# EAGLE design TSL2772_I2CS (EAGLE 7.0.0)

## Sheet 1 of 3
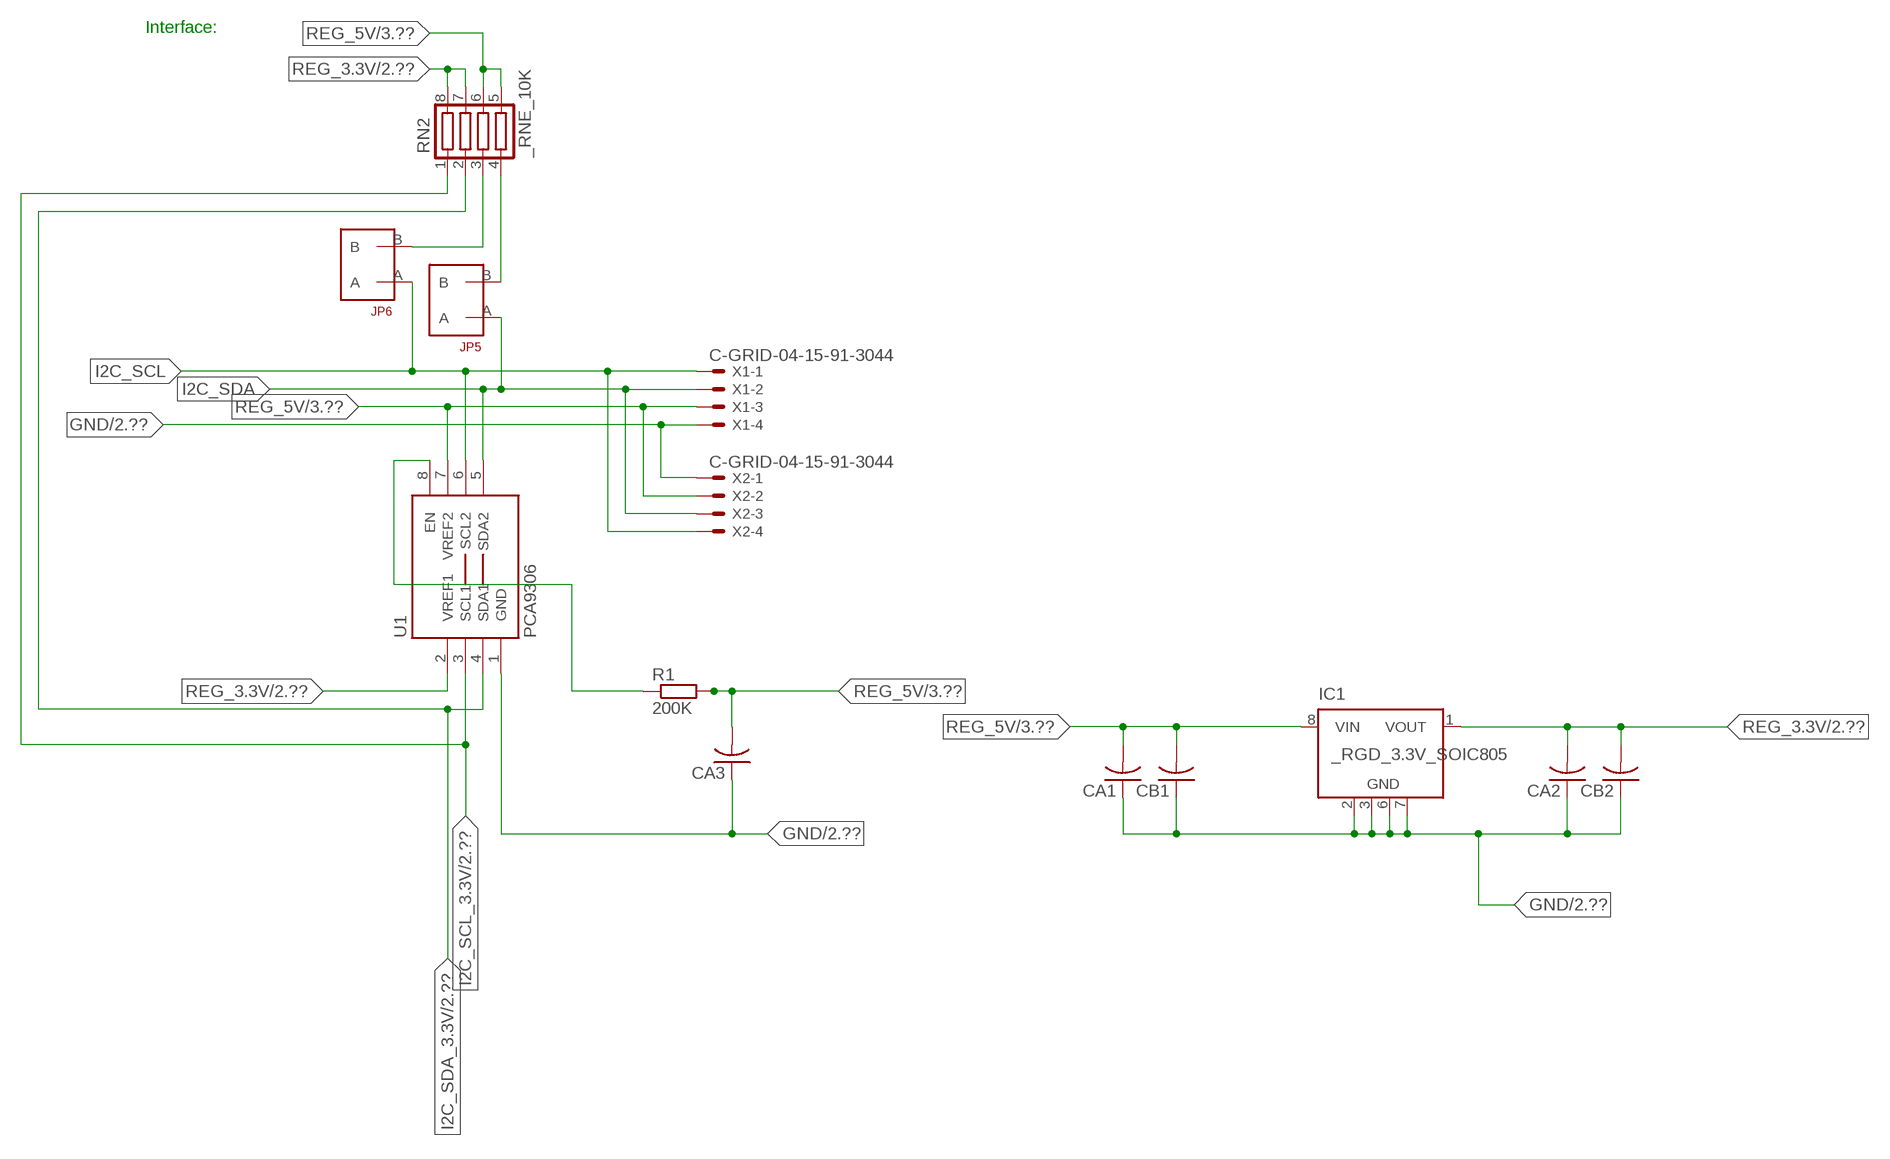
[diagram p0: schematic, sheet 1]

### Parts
CA1  CC1206KRX7R9BB104  [.1UF]
CA2  CC1206KRX7R9BB104  [.1UF]
CA3  CC1206KRX7R9BB104  [.1UF]
CB1  TMK316F106ZL-TC1206K  [TMK316F106ZL-T]
CB2  TMK316F106ZL-TC1206K  [TMK316F106ZL-T]
IC1  _RGD_3.3V_SOIC805  [_RGC_3.3V_SOIC8]
JP5  JUMPER_1X2_2MM  [JUMPER_1X2_2MM]
JP6  JUMPER_1X2_2MM  [JUMPER_1X2_2MM]
R1  200K  RESISTOR_SMT-0603  [R603]
RN2  _RNE_10K  [RNE]
U1  PCA9306  PCA9306_NCD  [PSOP-8]
X1  C-GRID-04-15-91-3044  [15-91-04]
X2  C-GRID-04-15-91-3044  [15-91-04]

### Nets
GND: CA1.1 CA2.1 CA3.1 CB1.1 CB2.1 IC1.2(GND) IC1.3(GND) IC1.6(GND) IC1.7(GND) U1.1(GND) X1.4 X2.1 ; also sheet 2,3
I2C_SCL: JP6.A U1.6(SCL2) X1.1 X2.4
I2C_SCL_3.3V: RN2.1 U1.3(SCL1) ; also sheet 2
I2C_SDA: JP5.A U1.5(SDA2) X1.2 X2.3
I2C_SDA_3.3V: RN2.2 U1.4(SDA1) ; also sheet 2
N$1: JP6.B RN2.3
N$2: JP5.B RN2.4
N$24: R1.1 U1.8(EN)
REG_3.3V: CA2.2 CB2.2 IC1.1(VOUT) RN2.7 RN2.8 U1.2(VREF1) ; also sheet 2
REG_5V: CA1.2 CA3.2 CB1.2 IC1.8(VIN) R1.2 RN2.5 RN2.6 U1.7(VREF2) X1.3 X2.2 ; also sheet 3
Unconnected: IC1.4(NC) IC1.5(NC)

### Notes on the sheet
- Interface:

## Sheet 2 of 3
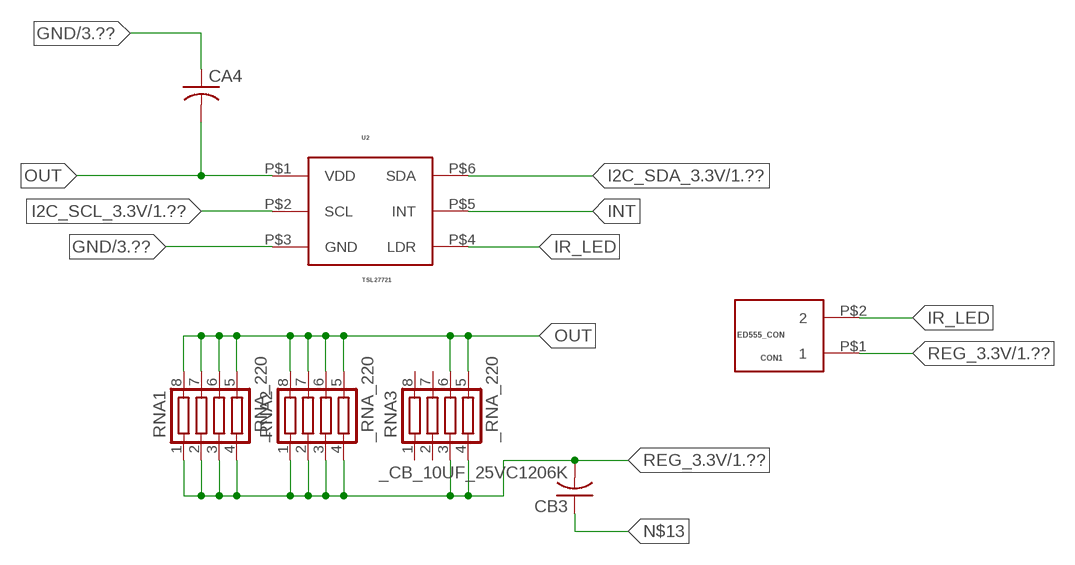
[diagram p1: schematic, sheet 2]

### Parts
CA4  _CA_.10UF_50VC1206K  [_CA_.1UF_50V]
CB3  _CB_10UF_25VC1206K  [_CB_10UF_25V]
CON1  ED555_CON  [ED555_CON]
RNA1  _RNA_220  [RNA]
RNA2  _RNA_220  [RNA]
RNA3  _RNA_220  [RNA]
U2  TSL27721  TSL2771  [TSL2771]

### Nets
GND: CA4.1 U2.P$3(GND) ; also sheet 1,3
I2C_SCL_3.3V: U2.P$2(SCL) ; also sheet 1
I2C_SDA_3.3V: U2.P$6(SDA) ; also sheet 1
INT: U2.P$5(INT)
IR_LED: CON1.P$2 U2.P$4(LDR)
N$13: CB3.1
OUT: CA4.2 RNA1.5 RNA1.6 RNA1.7 RNA1.8 RNA2.5 RNA2.6 RNA2.7 RNA2.8 RNA3.5 RNA3.6 U2.P$1(VDD)
REG_3.3V: CB3.2 CON1.P$1 RNA1.1 RNA1.2 RNA1.3 RNA1.4 RNA2.1 RNA2.2 RNA2.3 RNA2.4 RNA3.3 RNA3.4 ; also sheet 1
Unconnected: RNA3.1 RNA3.2 RNA3.7 RNA3.8

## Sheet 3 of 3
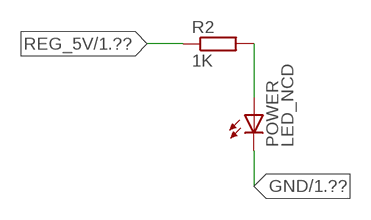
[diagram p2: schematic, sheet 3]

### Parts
POWER  LED_NCD  [CHIPLED_0603]
R2  1K  RESISTOR_SMT-0402  [R402]

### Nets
GND: POWER.C ; also sheet 1,2
N$4: POWER.A R2.2
REG_5V: R2.1 ; also sheet 1

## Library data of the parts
CA1-CA3 = NCD_ULTIMATE_LIBRARY:CC1206KRX7R9BB104: Capacitor CA .1uF 50V SMT C1206K CC1206KRX7R9BB104
CA4 = NCD_ULTIMATE_LIBRARY:_CA_.10UF_50V: Capacitor .1uF SMT
CB1 CB2 = NCD_ULTIMATE_LIBRARY:TMK316F106ZL-T: Capacitor CB 10uF SMT 1206 TMK316F106ZL-T
CB3 = NCD_ULTIMATE_LIBRARY:_CB_10UF_25V: Capacitor 10uF SMT
CON1 = NCD_ULTIMATE_bhaskar:ED555_CON: Digikey ED1514-ND/ ED555/2DS NCD CON
IC1 = NCD_ULTIMATE_LIBRARY:_RGD_3.3V_SOIC8: Regulator Linear 3.3V Chip Positive VOLTAGE REGULATOR Digikey 497-1199-2-ND/L78L33ACD13TR
JP5 JP6 = NCD_ULTIMATE_CONNECTORS:JUMPER_1X2_2MM
POWER = NCD_ULTIMATE_LIBRARY:LED_NCD: LED Digikey 754-1132-2-ND/APT2012SRCPRV
R1 R2 = NCD_ULTIMATE_LIBRARY:RESISTOR_SMT: NCD Resistor
RN2 = NCD_ULTIMATE_LIBRARY:_RNE_10K: Resistor Array RNE SMT 10K x 4 Single Resistor Source: http://www.ctscorp.com/components/Datasheets/CTSChipArrayDs.pdf Digikey 742C083103JPTR-ND/742C083103JP; OC_FARNELL: unknown; OC_NEWARK: unknown
RNA1-RNA3 = NCD_ULTIMATE_LIBRARY:_RNA_220: Resistor Array RNA SMT 220 x 4 Single Resistor Source: http://www.ctscorp.com/components/Datasheets/CTSChipArrayDs.pdf Digikey 742C083221JPTR-ND/742C083221JP; OC_FARNELL: unknown; OC_NEWARK: unknown
U1 = NCD_ULTIMATE_LIBRARY:PCA9306_NCD: NCD Bidirectional I2C level shifter. NOT compatible with all available part number pinout schemes- DOUBLE CHECK!!!; PROD_ID: IC-10023
U2 = NCD_ULTIMATE_bhaskar:TSL2771
X1 X2 = NCD_ULTIMATE_CONNECTORS:C-GRID-04: CONNECTOR 4-Pos I2C wire to board 2.54 mm (0.100") pitch header Digikey WM1342-ND/0015912045; OC_FARNELL: unknown; OC_NEWARK: unknown

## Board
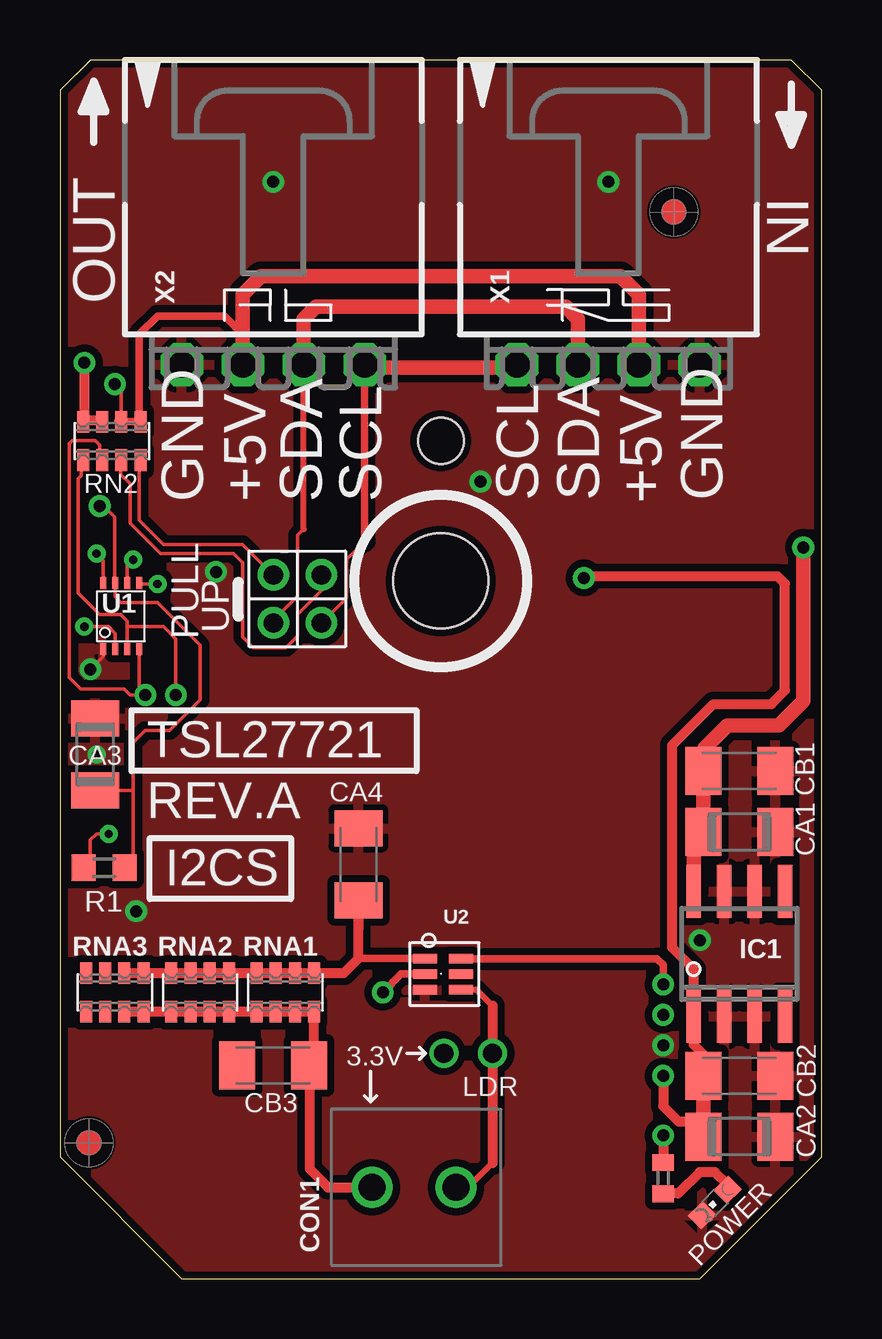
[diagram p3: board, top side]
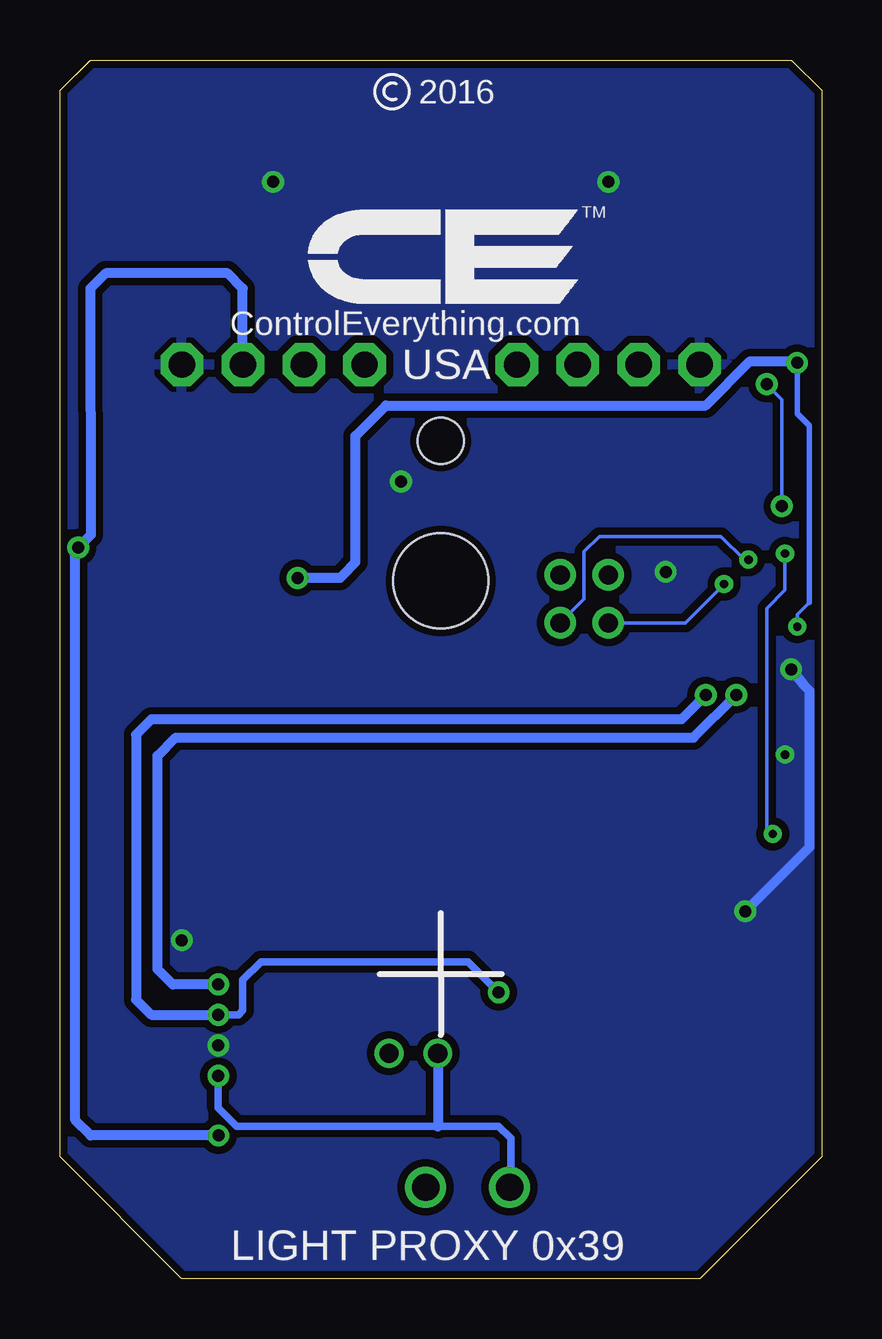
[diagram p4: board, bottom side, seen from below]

Size 31.75 x 50.8 mm. Coordinates in mm from the lower left corner, seen from the top.
Outline: 48 segments
Copper layers (1*16): Top 0.035mm / dielectric 1.5mm / Bottom 0.035mm
Design rules "default": minimum track width 5mil, minimum drill 24mil, track to track 5mil, track to pad 5mil, pad to pad 5mil, via to via 5mil, smd to smd 5mil, copper to edge 10mil, drill to drill 8mil, minimum pad ring 10mil, minimum via ring 8mil, stop-mask expansion 2mil, vias tented up to drill 0mil, thermal gap 10mil
Holes 3.96 mm at 15.88,29.08
Holes 1.91 mm at 15.88,34.93

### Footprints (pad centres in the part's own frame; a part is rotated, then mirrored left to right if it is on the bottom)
.1UF = smd 1.5 x 2: 1 -1.5,0; 2 1.5,0
_CA_.1UF_50V = smd 1.5 x 2: 1 -1.5,0; 2 1.5,0
TMK316F106ZL-T = smd 1.5 x 2: 1 -1.5,0; 2 1.5,0
_CB_10UF_25V = smd 1.5 x 2: 1 -1.5,0; 2 1.5,0
ED555_CON = drill 1.143: P$1 0,3.5; P$2 0,0
_RGC_3.3V_SOIC8 = smd 0.6 x 2.2: 1 -1.905,-2.6; 2 -0.635,-2.6; 3 0.635,-2.6; 4 1.905,-2.6; 5 1.905,2.6; 6 0.635,2.6; 7 -0.635,2.6; 8 -1.905,2.6
JUMPER_1X2_2MM = drill 0.8: A 0,2; B 0,0
CHIPLED_0603 = smd 0.8 x 0.876: A 0,-0.75; C 0,0.75
R603 = smd 1 x 1.1: 1 -0.85,0; 2 0.85,0
R402 = smd 0.7 x 0.9: 1 -0.65,0; 2 0.65,0
RNE = smd 0.5 x 0.9: 1 -1.2,-0.8; 2 -0.4,-0.8; 3 0.4,-0.8; 4 1.2,-0.8; 5 1.2,0.8; 6 0.4,0.8; 7 -0.4,0.8; 8 -1.2,0.8
RNA = smd 0.5 x 0.9: 1 -1.2,-0.8; 2 -0.4,-0.8; 3 0.4,-0.8; 4 1.2,-0.8; 5 1.2,0.8; 6 0.4,0.8; 7 -0.4,0.8; 8 -1.2,0.8
PSOP-8 = smd 0.25 x 0.5: 1 -0.73,-1.37; 2 -0.23,-1.37; 3 0.27,-1.37; 4 0.77,-1.37; 5 0.77,1.38; 6 0.27,1.38; 7 -0.23,1.38; 8 -0.73,1.38
TSL2771 = smd 1 x 0.4: P$1 -0.65,0.65; P$2 -0.65,0; P$3 -0.65,-0.65; P$4 0.85,-0.65; P$5 0.85,0; P$6 0.85,0.65
15-91-04 = drill 1.1 pad 1.778 octagon: 1 -3.81,-7.62; 2 -1.27,-7.62; 3 1.27,-7.62; 4 3.81,-7.62

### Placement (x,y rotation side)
CA1  28.32,18.62 180 top
CA2  28.32,5.92 180 top
CA3  1.46,21.86 270 top
CA4  12.45,17.27 270 top
CB1  28.32,21.16 180 top
CB2  28.32,8.46 180 top
CB3  8.89,8.89 0 top
CON1  16.51,3.81 90 top
IC1  28.32,13.54 0 top
JP5  8.89,29.34 180 top
JP6  10.9,29.34 180 top
POWER  27.3,3.18 135 top
R1  1.84,17.13 0 top
R2  25.15,4.19 270 top
RN2  2.16,34.93 0 top
RNA1  9.4,11.94 0 top
RNA2  5.84,11.94 0 top
RNA3  2.29,11.94 0 top
U1  2.54,27.61 0 top
U2  15.88,12.7 0 top
U$5  [VISION_REF10]  1.21,5.66 90 top
U$28  [VISION_REF10]  25.59,44.46 90 top
X1  22.86,45.72 0 top
X2  8.89,45.72 0 top

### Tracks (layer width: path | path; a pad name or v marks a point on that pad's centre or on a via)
GND  (via drill 0.35, 0.5)
  Top 0.152: CA3.1 1.52,23.42 1.52,23.62 | v1.27,25.4 1.81,25.94 U1.1
  Bottom 0.406: v1.27,25.4 0.76,24.77 0.51,24.51 0.51,17.99 v3.18,15.32
  other vias: 8.89,45.72 22.86,45.72 25.15,9.73 17.53,33.22 26.67,14.11 6.5,29.46 1.52,21.84
  pour Bottom (isolate 0.305): -0.64,5.08 -0.64,49.53 1.27,51.44 30.48,51.44 32.38,49.53 32.38,5.08 26.67,-0.63 5.08,-0.63
  pour Top (isolate 0.305): 4.45,-1.27 -1.27,4.45 -1.27,50.17 0.64,52.07 31.11,52.07 33.02,50.17 33.02,4.45 27.3,-1.27
I2C_SCL  (via drill 0.35)
  Top 0.152: 12.7,30.73 11.94,29.97 11.94,28.38 JP6.A | v3.05,29.97 2.81,29.73 U1.6
  Top 0.305: 12.7,30.73 X2.4
  Top 0.406: X2.4 12.7,37.97 | 19.05,37.97 X1.1
  Top 0.61: 12.7,37.97 19.05,37.97
  Bottom 0.152: JP6.A 9.91,28.33 9.91,30.3 9.27,30.94 4.19,30.94 3.23,29.97 v3.05,29.97
I2C_SCL_3.3V  (via drill 0.5)
  Top 0.152: RN2.1 0.89,34.07 0.89,33.48 0.77,33.35 0.77,28.59 1.67,27.69 2.54,27.69 2.81,27.42 2.81,27.18 | 2.81,27.18 U1.3 | v4.83,24.33 v4.83,24.34 4.83,26.67 4.32,27.18 2.81,27.18
  Top 0.305: U2.P$2 14.22,12.7 v13.46,11.94
  Bottom 0.305: v13.46,11.94 14.73,13.21 23.37,13.21 24.13,12.45 24.13,11.18 24.31,11 v25.15,11
  Bottom 0.406: v4.83,24.33 5.84,23.32 27.94,23.32 28.58,22.68 28.58,11.63 27.94,11 v25.15,11
I2C_SDA  (via drill 0.35)
  Top 0.152: JP5.A 8.89,27.44 9.91,28.45 9.91,30.99 10.16,31.24 | U1.5 3.34,28.96 v4.06,28.96
  Top 0.254: 10.16,31.24 10.16,31.25 X2.3
  Top 0.61: X2.3 10.16,40.01 10.67,40.51 21.09,40.51 21.59,40.01 X1.2
  Bottom 0.152: v4.06,28.96 5.68,27.34 JP5.A
I2C_SDA_3.3V  (via drill 0.5)
  Top 0.152: RN2.2 1.65,34.14 1.65,34.75 1.46,34.94 0.51,34.94 0.38,34.81 0.38,26.37 0.38,26.36 0.38,25.07 0.86,24.59 2.67,24.59 2.92,24.33 v3.56,24.33 3.31,24.58 U1.4
  Top 0.305: U2.P$6 17.12,13.34 24.89,13.34 25.15,13.08 v25.15,12.27
  Bottom 0.406: v25.15,12.27 27.05,12.27 27.69,12.9 27.69,21.79 26.93,22.56 5.34,22.56 v3.56,24.33
IR_LED  (via drill 0.8)
  Top 0.254: 18.03,11.38 17.36,12.05 U2.P$4 | 18.03,4.83 17.02,3.81 CON1.P$2
  Top 0.406: 18.03,11.38 v18.03,9.4 18.03,4.83
N$1
  Top 0.152: JP6.B 10.92,29.31 10.92,28.7 9.91,27.69 9.91,26.8 9.42,26.31 8.06,26.31 7.62,26.75 7.62,29.84 7.24,30.23 4.19,30.23 2.92,31.5 2.92,33.15 2.54,33.53 2.54,34.1 RN2.3
  Top 0.305: 2.54,34.02 RN2.3
N$2
  Top 0.152: JP5.B 7.62,30.61 4.32,30.61 3.3,31.62 3.3,34.07 RN2.4
  Top 0.305: 3.37,33.88 RN2.4
N$4
  Top 0.406: POWER.A 27.84,3.92 27.3,4.45 26.67,4.45 25.78,3.56 25.16,3.56 R2.2
N$24  (via drill 0.35)
  Top 0.152: R1.1 1.27,17.41 1.27,18.29 1.52,18.54 v2.03,18.54 | v1.52,30.23 1.81,29.94 U1.8
  Bottom 0.152: v2.03,18.54 2.29,18.8 2.29,27.94 1.52,28.7 v1.52,30.23
OUT
  Top 0.305: 12.44,13.35 U2.P$1
  Top 0.406: RNA3.6 RNA3.5 RNA2.8 RNA2.7 RNA2.6 RNA2.5 RNA1.8 RNA1.7 RNA1.6 RNA1.5 11.84,12.74 12.45,13.34 CA4.2 12.44,13.35
REG_3.3V  (via drill 0.35, 0.5, 0.8)
  Top 0.152: v1.02,27.18 2.03,27.18 2.31,26.9 U1.2
  Top 0.406: CB2.2 26.82,9.35 26.42,9.75 26.42,10.36 | v25.15,8.46 25.15,7.19 25.78,6.55 26.82,6.55 | IC1.1 26.42,12.9 25.53,13.79 25.53,22.24 27.24,23.95 29.66,23.95 30.23,24.52 30.23,28.97 29.91,29.29 21.92,29.29 v21.84,29.21 | 26.52,5.62 CA2.2 | v1.02,38.18 1.02,35.78 | 1.02,35.78 RN2.8 | 1.02,35.78 1.71,35.78 RN2.7 | RNA3.3 RNA3.4 RNA2.1 RNA2.2 RNA2.3 RNA2.4 RNA1.1 RNA1.2 RNA1.3 RNA1.4 10.6,8.89 | CB3.2 10.6,8.89 | 10.6,8.89 10.41,8.71 10.41,4.57 11.18,3.81 CON1.P$1
  Top 0.61: CB2.2 26.82,6.55 CA2.2 | 26.42,10.36 IC1.1
  Bottom 0.152: 0.51,28.19 1.02,27.69 v1.02,27.18
  Bottom 0.229: 0.51,28.19 0.51,35.56 1.02,36.07 v1.02,38.18
  Bottom 0.305: CON1.P$1 12.95,3.87 12.95,5.84 13.46,6.35 16,6.35 24.38,6.35 25.15,7.12 v25.15,8.46
  Bottom 0.406: v1.02,38.18 1.08,38.24 2.99,38.24 4.83,36.4 18.16,36.4 19.43,35.13 19.43,29.87 19.94,29.34 20.07,29.21 v21.84,29.21 | v16,9.4 16,6.35
REG_5V  (via drill 0.5)
  Top 0.152: RN2.6 2.56,37.01 v2.29,37.29 | R1.2 3.05,17.49 3.05,20.36 | 3.05,20.36 3.05,22.35 3.56,22.86 4.57,22.86 5.84,24.13 5.84,26.42 4.06,28.19 2.54,28.19 2.31,28.43 U1.7 2.29,29.01 2.29,31.75 1.83,32.21 v1.65,32.21 | CA3.2 3.05,20.36
  Top 0.305: 7.62,39.37 7.5,39.37 | 2.42,35.74 RN2.6 RN2.5 3.31,35.8 3.31,39.37 4.07,40.13 6.86,40.13 7.62,39.37 | X2.2 7.62,39.37
  Top 0.406: v25.15,5.97 R2.1
  Top 0.61: X2.2 7.62,41.02 8.38,41.78 23.37,41.78 24.13,41.02 X1.3 | IC1.8 26.42,18.21 CA1.2 CB1.2 26.86,21.2 26.86,22.11 27.82,23.06 29.98,23.06 30.99,24.08 v30.99,30.48
  Bottom 0.152: v1.65,32.21 1.65,36.65 v2.29,37.29
  Bottom 0.406: X1.3 24.13,41.28 24.77,41.91 29.84,41.91 30.48,41.27 30.47,31 v30.99,30.48 31.11,30.36 31.11,6.6 30.48,5.97 v25.15,5.97

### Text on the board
tNames: IN | OUT | GND | +5V | SDA | SCL | SCL | SDA | +5V | GND | PULL | UP | TSL27721 | REV.A | I2CS | 3.3V | LDR
bNames: 2016 | TM | ControlEverything.com | USA | LIGHT PROXY 0x39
